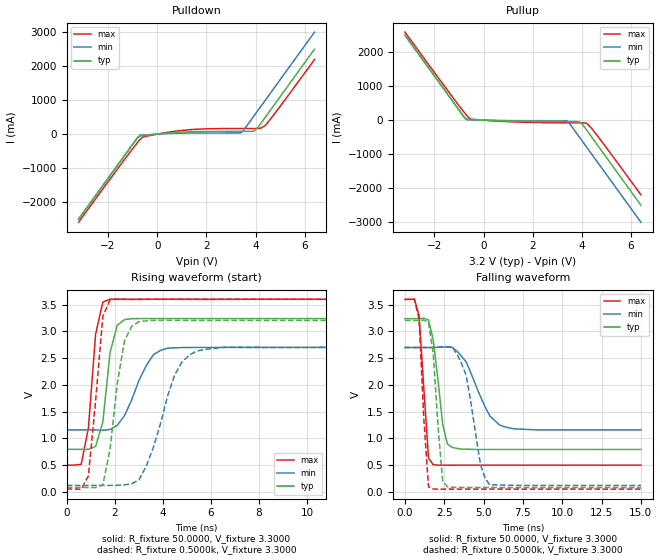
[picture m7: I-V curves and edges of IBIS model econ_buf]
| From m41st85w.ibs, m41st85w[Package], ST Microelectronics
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|   Model econ_buf
[Model]   econ_buf
Model_type   Output
Polarity   Non-Inverting
Enable   Active-Low
Vmeas =   1.5000V
Cref =  50.0000pF
Rref =   0.3330k
Vref =   1.7300V
C_comp   7.8900pF   7.4700pF   8.3400pF
[Temperature Range]   27.0000   85.0000   -40.0000
[Voltage Range]   3.2000V   2.7000V   3.6000V
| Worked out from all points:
|   slope of the pulldown table from 0 to 0.48 V, typ, clamps not added: 14.3 ohm
|   slope of the pullup table from 0 to 0.48 V, typ, clamps not added: 36.1 ohm
|   rising waveform, R_fixture 50.0000, V_fixture 3.3000: 20-80 % time 403ps typ, 911ps min, 346ps max; typ from 0.793 V to 3.24 V
|   rising waveform, R_fixture 0.5000k, V_fixture 3.3000: 20-80 % time 549ps typ, 1.05ns min, 427ps max; typ from 0.081 V to 3.21 V
|   falling waveform, R_fixture 50.0000, V_fixture 3.3000: 20-80 % time 556ps typ, 1.37ns min, 419ps max; typ from 3.24 V to 0.793 V
|   falling waveform, R_fixture 0.5000k, V_fixture 3.3000: 20-80 % time 453ps typ, 849ps min, 388ps max; typ from 3.21 V to 0.081 V
[Pulldown]
| voltage   I(typ)   I(min)   I(max)
-3.2V     -2.5A      -2.5A      -2.59A
-900mV    -200mA     -200mA     -336mA
-700mV    -62.45mA   -32.66mA   -159.6mA
-500mV    -39.89mA   -23.29mA   -67.65mA
900mV     54.81mA    27.57mA    99.89mA
3.4V      81.17mA    34.99mA    165.9mA
3.5V      81.34mA    100mA      166.2mA
3.9V      85.33mA    500mA      167.5mA
4V        121.5mA    600mA      167.8mA
4.2V      300mA      800mA      168.7mA
4.4V      500mA      1A         256.9mA
6.4V      2.5A       3A         2.194A
[Pullup]
| voltage   I(typ)   I(min)   I(max)
-3.2V     2.5A       2.5A       2.589A
-900mV    200mA      200mA      332.4mA
-700mV    40.84mA    13.48mA    150.9mA
-500mV    16.26mA    9.073mA    29.82mA
-300mV    9.594mA    5.335mA    16.42mA
1.4V      -30.1mA    -14.05mA   -55.75mA
3.4V      -38.98mA   -17.33mA   -78.6mA
3.9V      -52.25mA   -500mA     -80.59mA
4V        -107.8mA   -600mA     -80.96mA
4.2V      -300mA     -800mA     -95mA
4.6V      -700mA     -1.2A      -429.4mA
6.4V      -2.5A      -3A        -2.193A
[Ramp]
| variable   typ   min   max
dV/dt_r   1.7392/0.5452n   1.3437/1.1489n   2.0422/0.2886n
dV/dt_f   1.8492/0.4055n   1.5128/0.8560n   2.1141/0.2331n
R_load = 0.3330k
[Rising Waveform]
R_fixture = 50.0000
V_fixture = 3.3000
V_fixture_min = 2.7000
V_fixture_max = 3.6000
| time   V(typ)   V(min)   V(max)
0s        793mV      1.158V     498.3mV
600ps     792.6mV    1.158V     512mV
900ps     792.5mV    1.158V     1.188V
1.2ns     847.7mV    1.157V     2.949V
1.5ns     1.306V     1.151V     3.548V
1.8ns     2.6V       1.164V     3.603V
2.4ns     3.219V     1.423V     3.599V
3.3ns     3.239V     2.353V     3.601V
4.2ns     3.239V     2.685V     3.6V
15ns      3.239V     2.7V       3.601V
[Rising Waveform]
R_fixture = 0.5000k
V_fixture = 3.3000
V_fixture_min = 2.7000
V_fixture_max = 3.6000
| time   V(typ)   V(min)   V(max)
0s        81.1mV     119mV      50.58mV
900ps     80.24mV    119mV      296.3mV
1.5ns     127.7mV    118.7mV    3.279V
1.8ns     793.9mV    118.4mV    3.586V
2.1ns     2.021V     119.9mV    3.604V
2.4ns     2.821V     128.8mV    3.601V
3ns       3.179V     220.4mV    3.598V
4.5ns     3.207V     2.197V     3.601V
5.4ns     3.204V     2.63V      3.6V
15ns      3.206V     2.7V       3.601V
[Falling Waveform]
R_fixture = 50.0000
V_fixture = 3.3000
V_fixture_min = 2.7000
V_fixture_max = 3.6000
| time   V(typ)   V(min)   V(max)
0s        3.239V     2.7V       3.6V
600ps     3.239V     2.7V       3.606V
900ps     3.24V      2.7V       3.296V
1.5ns     3.214V     2.7V       633.6mV
1.8ns     2.843V     2.7V       506.1mV
2.4ns     1.264V     2.708V     498.6mV
3ns       832.1mV    2.704V     498.1mV
3.9ns     797.6mV    2.426V     498.4mV
6ns       793mV      1.255V     498.2mV
15ns      793mV      1.158V     498.3mV
[Falling Waveform]
R_fixture = 0.5000k
V_fixture = 3.3000
V_fixture_min = 2.7000
V_fixture_max = 3.6000
| time   V(typ)   V(min)   V(max)
0s        3.206V     2.7V       3.6V
900ps     3.207V     2.7V       3.231V
1.5ns     3.166V     2.7V       93.45mV
1.8ns     2.588V     2.7V       53.17mV
2.4ns     197.3mV    2.712V     50.63mV
2.7ns     93.96mV    2.717V     51.53mV
3.9ns     81.4mV     2.173V     49.64mV
4.8ns     81.08mV    513.3mV    50.77mV
5.4ns     81.25mV    123.5mV    51.45mV
15ns      81.21mV    119mV      51.28mV
